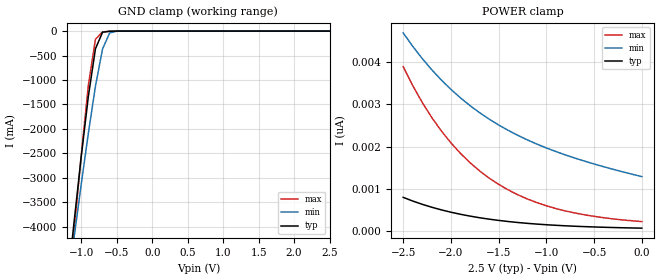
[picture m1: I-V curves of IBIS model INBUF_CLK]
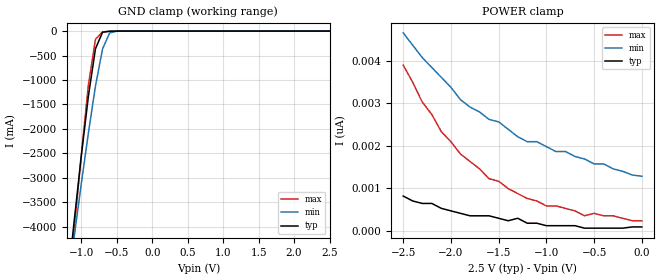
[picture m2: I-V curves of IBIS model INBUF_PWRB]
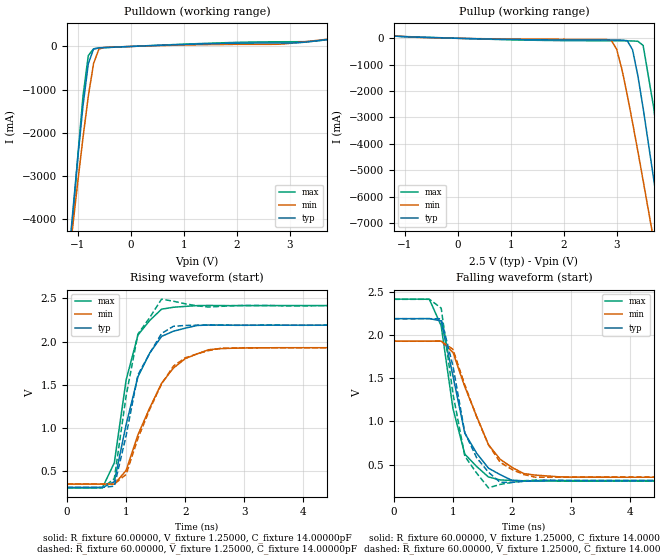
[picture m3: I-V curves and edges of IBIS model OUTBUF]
| IBIS file cspt857_mlf_2p5.ibs created by s2ibis2 version 1.2
| North Carolina State University Electronics Research Laboratory  1995
[IBIS ver]   2.1
[File name]   cspt857c_mlf_2p5.ibs
[File Rev]   1.0
[Date]   Friday, May 09, 2003
[Source]   IDT
[Notes]   1. Temp typ=25C, min=0C, max=100C
   2. IDT's 2.0v C11.5 process
   3. Ramp rate based on 50 ohm load
READ THESE TERMS AND CONDITIONS CAREFULLY BEFORE USING THIS IBIS MODEL.  BY
USING THIS IBIS MODEL, YOU ARE ACCEPTING AND AGREEING TO THESE TERMS AND
CONDITIONS OF USE.
Integrated Device Technology, Inc. ("IDT") hereby grants the user of this
IBIS model ("User") a non-exclusive, nontransferable license to use this
IBIS model under the following terms: The User is granted this license only
to use the IBIS model for demonstration purposes only and is not granted
rights to sell, copy (except as needed to run the IBIS model), rent, lease
or sub-license (except for demonstration) the IBIS model in whole or in
part, or in modified form to anyone. The User may modify the IBIS model to
suit its specific applications, but  rights to derivative works and such
modifications shall belong to IDT.
THIS IBIS MODEL IS PROVIDED ON AN AS IS" BASIS AND IDT  MAKES ABSOLUTELY NO
WARRANTY WITH RESPECT TO THE INFORMATION CONTAINED HEREIN.  IDT DISCLAIMS
AND USER WAIVES ALL WARRANTIES, EXPRESS AND IMPLIED, INCLUDING WARRANTIES OF
MERCHANTABILITY AND FITNESS FOR A PARTICULAR PURPOSE.  THE ENTIRE RISK AS TO
QUALITY AND PERFORMANCE IS WITH THE USER  ACCORDINGLY, IN NO EVENT SHALL IDT
BE LIABLE FOR ANY DIRECT OR INDIRECT DAMAGES, WHETHER IN CONTRACT OR TORT,
INCLUDING ANY LOST PROFITS OR OTHER INCIDENTAL, CONSEQUENTIAL, EXEMPLARY, OR
PUNITIVE DAMAGES ARISING OUT OF THE USE OR APPLICATION OF THE  IBIS MODEL,
WHETHER OR NOT IDT HAD NOTICE OF SUCH DAMAGES.
IDT reserves the right to make changes without notice to any product herein
to improve
reliability, function, or design. IDT does not convey any license under
patent rights or any other intellectual property rights, including those of
third parties. IDT is not obligated
to provide maintenance or support for the licensed IBIS model.
This model is for the 2.5V Phase Locked Loop Differential 1:10 SDRAM Clock
Driver
[Copyright]
Copyright 2002, Integrated Device Technology, Inc. All rights reserved.
|   Component CPST857C
[Component]   CPST857C
[Manufacturer]   Integrated Device Technology Inc.
[Package]
| variable   typ   min   max
R_pkg   86.00000m   61.00000m   0.11300
L_pkg   2.10000nH   1.50000nH   2.70000nH
C_pkg   0.20000pF   0.16000pF   0.24000pF
[Pin]  signal_name   model_name   R_pin   L_pin   C_pin
1   GND   GND
2   _Y2_   OUTBUF
3   Y2   OUTBUF
4   VDDQ   POWER
5   CLK   INBUF_CLK
6   _CLK_   INBUF_CLK
7   VDDQ   POWER
8   AVDD   POWER
9   AGND   GND
10   GND   GND
11   _Y3_   OUTBUF
12   Y3   OUTBUF
13   VDDQ   POWER
14   Y4   OUTBUF
15   _Y4_   OUTBUF
16   _Y9_   OUTBUF
17   Y9   OUTBUF
18   VDDQ   POWER
19   Y8   OUTBUF
20   _Y8_   OUTBUF
21   FBOUT   OUTBUF
22   _FBOUT_   OUTBUF
23   VDDQ   POWER
24   VDDQ   POWER
25   _FBIN_   INBUF_FBIN
26   FBIN   INBUF_FBIN
27   _PWRDWN_   INBUF_PWRB
28   VDDQ   POWER
29   Y7   OUTBUF
30   _Y7_   OUTBUF
31   _Y6_   OUTBUF
32   Y6   OUTBUF
33   VDDQ   POWER
34   Y5   OUTBUF
35   _Y5_   OUTBUF
36   _Y0_   OUTBUF
37   Y0   OUTBUF
38   VDDQ   POWER
39   Y1   OUTBUF
40   _Y1_   OUTBUF
| in   in   dummy_model
[Diff Pin]  inv_pin  vdiff   tdelay_typ  tdelay_min  tdelay_max
5   6   1.00000V  NA  |CLK<P:N> Clock Input  Pair
26   25   1.00000V  NA  |FBIN<P:N> FBIN Input  Pair
3   2   0.000V   NA  |Y2<P:N> Ouput  Pair
12   11   0.000V   NA  |Y3<P:N> Ouput  Pair
14   15   0.000V   NA  |Y4<P:N> Ouput  Pair
17   16   0.000V   NA  |Y9<P:N> Ouput  Pair
19   20   0.000V   NA  |Y8<P:N> Ouput  Pair
21   22   0.000V   NA  |FBOUT<P:N> Ouput  Pair
29   30   0.000V   NA  |Y7<P:N> Ouput  Pair
32   31   0.000V   NA  |Y6<P:N> Ouput  Pair
34   35   0.000V   NA  |Y5<P:N> Ouput  Pair
37   36   0.000V   NA  |Y0<P:N> Ouput  Pair
39   40   0.000V   NA  |Y1<P:N> Ouput  Pair
| Models and submodels in the file (4): INBUF_CLK (Input), INBUF_PWRB (Input), INBUF_FBIN (Input), OUTBUF (Output)
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|   Model INBUF_CLK
[Model]   INBUF_CLK
Model_type   Input
Polarity   Non-Inverting
Vinl =  0.80000V
Vinh =  2.00000V
C_comp   3.50000pF   3.50000pF   3.50000pF
[Temperature Range]   25.00000   100.00000   0.000
[Voltage Range]   2.50000V   2.30000V   2.70000V
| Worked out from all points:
|   GND clamp passes 1 mA (typ) near -0.52 V on its own axis
[GND_clamp]
| voltage   I(typ)   I(min)   I(max)
-2.5V     -23.89A    -20.36A    -27.98A
-1.2V     -5.248A    -5.316A    -5.713A
-1.1V     -3.884A    -4.209A    -4.089A
-1V       -2.564A    -3.127A    -2.526A
-900mV    -1.335A    -2.086A    -1.108A
-800mV    -361.3mA   -1.127A    -168.2mA
-700mV    -23.9mA    -365.3mA   -14.69mA
-600mV    -2.784mA   -39.09mA   -5.291mA
-500mV    -459.2uA   -2.159mA   -1.358mA
2.5V      71.27pA    1.402nA    195.1pA
[POWER_clamp]
| voltage   I(typ)   I(min)   I(max)
-2.5V     798.8pA    4.684nA    3.887nA
-2.4V     712pA      4.366nA    3.439nA
-2.3V     634.4pA    4.076nA    3.039nA
-2.2V     565pA      3.811nA    2.683nA
-2V       448.2pA    3.35nA     2.086nA
-1.8V     356pA      2.967nA    1.618nA
-1.7V     317.8pA    2.8nA      1.425nA
-1.5V     254.3pA    2.509nA    1.106nA
-1.2V     185.1pA    2.157nA    761.7pA
-900mV    138.7pA    1.881nA    534.7pA
-500mV    99.57pA    1.587nA    349.9pA
0V        71.27pA    1.288nA    226.3pA
|   Model INBUF_PWRB
[Model]   INBUF_PWRB
Model_type   Input
Polarity   Non-Inverting
Vinl =  0.80000V
Vinh =  2.00000V
C_comp   3.50000pF   3.50000pF   3.50000pF
[Temperature Range]   25.00000   100.00000   0.000
[Voltage Range]   2.50000V   2.30000V   2.70000V
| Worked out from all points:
|   GND clamp passes 1 mA (typ) near -0.52 V on its own axis
[GND_clamp]
| voltage   I(typ)   I(min)   I(max)
-2.5V     -23.88A    -20.35A    -27.98A
-1.2V     -5.247A    -5.316A    -5.712A
-1.1V     -3.884A    -4.209A    -4.088A
-1V       -2.564A    -3.127A    -2.526A
-900mV    -1.335A    -2.086A    -1.108A
-800mV    -361.3mA   -1.126A    -168.2mA
-700mV    -23.9mA    -365.3mA   -14.69mA
-600mV    -2.784mA   -39.09mA   -5.291mA
-500mV    -459.2uA   -2.159mA   -1.358mA
2.5V      87.31pA    1.397nA    232.8pA
[POWER_clamp]
| voltage   I(typ)   I(min)   I(max)
-2.5V     814.9pA    4.657nA    3.9nA
-2.3V     640.3pA    4.075nA    3.027nA
-2.1V     523.9pA    3.609nA    2.328nA
-1.9V     407.5pA    3.085nA    1.804nA
-1.6V     349.2pA    2.619nA    1.222nA
-1.5V     291pA      2.561nA    1.164nA
-1.3V     291pA      2.212nA    873.1pA
-1.2V     174.6pA    2.095nA    756.7pA
-1V       116.4pA    1.979nA    582.1pA
-600mV    58.21pA    1.688nA    349.2pA
-500mV    58.21pA    1.572nA    407.5pA
0V        87.31pA    1.281nA    232.8pA
|   Model OUTBUF
[Model]   OUTBUF
Model_type   Output
Polarity   Non-Inverting
Vmeas =  1.25000V
C_comp   3.50000pF   3.50000pF   3.50000pF
[Temperature Range]   25.00000   100.00000   0.000
[Voltage Range]   2.50000V   2.30000V   2.70000V
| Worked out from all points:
|   slope of the pulldown table from 0 to 0.375 V, typ, clamps not added: 20.3 ohm
|   slope of the pullup table from 0 to 0.375 V, typ, clamps not added: 20 ohm
|   rising waveform, R_fixture 60.00000, V_fixture 1.25000, C_fixture 14.00000pF: 20-80 % time 468ps typ, 633ps min, 341ps max; typ from 0.315 V to 2.19 V
|   rising waveform, R_fixture 60.00000, V_fixture 1.25000, C_fixture 14.00000pF: 20-80 % time 436ps typ, 602ps min, 308ps max; typ from 0.316 V to 2.19 V
|   falling waveform, R_fixture 60.00000, V_fixture 1.25000, C_fixture 14.00000pF: 20-80 % time 441ps typ, 581ps min, 335ps max; typ from 2.19 V to 0.315 V
|   falling waveform, R_fixture 60.00000, V_fixture 1.25000, C_fixture 14.00000pF: 20-80 % time 388ps typ, 552ps min, 299ps max; typ from 2.19 V to 0.316 V
[Pulldown]
| voltage   I(typ)   I(min)   I(max)
-2.5V     -24.02A    -20.48A    -28.11A
-1.3V     -6.698A    -6.489A    -7.44A
-1.1V     -3.936A    -4.25A     -4.147A
-1V       -2.612A    -3.164A    -2.58A
-900mV    -1.378A    -2.12A     -1.157A
-800mV    -400.3mA   -1.157A    -211.8mA
-700mV    -58.29mA   -391.9mA   -53.12mA
-600mV    -32.51mA   -62.11mA   -38.49mA
-500mV    -25.4mA    -21.54mA   -29.24mA
2.8V      81.34mA    52.63mA    108.7mA
3.2V      89.68mA    97.53mA    110.8mA
5V        376.9mA    361.1mA    377.2mA
[Pullup]
| voltage   I(typ)   I(min)   I(max)
-2.5V     286.8mA    273.7mA    294mA
-900mV    50.69mA    50.88mA    59.76mA
2.9V      -64.27mA   -81.77mA   -93.6mA
3V        -64.95mA   -412.9mA   -93.85mA
3.2V      -91.83mA   -2.145A    -95.98mA
3.3V      -434.2mA   -3.192A    -101.2mA
3.4V      -1.414A    -4.28A     -112.7mA
3.5V      -2.65A     -5.394A    -270mA
3.7V      -5.347A    -7.664A    -2.64A
3.9V      -8.156A    -9.969A    -5.841A
4.1V      -11.01A    -12.29A    -9.193A
5V        -24.08A    -22.88A    -24.72A
[Ramp]
| variable   typ   min   max
dV/dt_r   1.04760/0.15068n   0.82920/0.17415n   1.21080/0.13672n
dV/dt_f   1.05510/0.13771n   0.87414/0.16331n   1.18398/0.13634n
R_load = 50.00000
[Rising Waveform]
R_fixture = 60.00000
V_fixture = 1.25000
V_fixture_min = 1.15000
V_fixture_max = 1.35000
C_fixture = 14.00000pF
| time   V(typ)   V(min)   V(max)
0s        315.1mV    354mV      310.2mV
600ps     314.6mV    354mV      313.6mV
800ps     380.5mV    352.7mV    599.6mV
1ns       1.042V     511.7mV    1.557V
1.2ns     1.595V     922.9mV    2.076V
1.4ns     1.869V     1.235V     2.245V
1.6ns     2.061V     1.518V     2.376V
2ns       2.155V     1.803V     2.408V
2.6ns     2.192V     1.919V     2.417V
10ns      2.191V     1.93V      2.417V
[Rising Waveform]
R_fixture = 60.00000
V_fixture = 1.25000
V_fixture_min = 1.15000
V_fixture_max = 1.35000
C_fixture = 14.00000pF
R_dut = 86.00000m
L_dut = 2.10000nH
C_dut = 0.20000pF
| time   V(typ)   V(min)   V(max)
0s        316.1mV    354.8mV    311.4mV
600ps     316mV      354.8mV    311.4mV
800ps     329.3mV    354.3mV    416.1mV
1ns       913.4mV    465.2mV    1.374V
1.2ns     1.617V     881.1mV    2.088V
1.6ns     2.095V     1.51V      2.491V
1.8ns     2.178V     1.718V     2.467V
2ns       2.187V     1.812V     2.438V
2.6ns     2.192V     1.923V     2.408V
10ns      2.19V      1.929V     2.415V
[Falling Waveform]
R_fixture = 60.00000
V_fixture = 1.25000
V_fixture_min = 1.15000
V_fixture_max = 1.35000
C_fixture = 14.00000pF
| time   V(typ)   V(min)   V(max)
0s        2.191V     1.93V      2.417V
600ps     2.192V     1.93V      2.415V
800ps     2.164V     1.931V     2.108V
1ns       1.526V     1.799V     1.147V
1.2ns     864.3mV    1.401V     621.2mV
1.6ns     459.2mV    731.7mV    356.9mV
1.8ns     383.4mV    560.5mV    322.2mV
2.2ns     311.3mV    396mV      312.7mV
2.8ns     315.2mV    358.3mV    310.2mV
10ns      315.1mV    354mV      310.2mV
[Falling Waveform]
R_fixture = 60.00000
V_fixture = 1.25000
V_fixture_min = 1.15000
V_fixture_max = 1.35000
C_fixture = 14.00000pF
R_dut = 86.00000m
L_dut = 2.10000nH
C_dut = 0.20000pF
| time   V(typ)   V(min)   V(max)
0s        2.19V      1.929V     2.415V
600ps     2.19V      1.929V     2.415V
800ps     2.189V     1.93V      2.313V
1ns       1.639V     1.835V     1.319V
1.2ns     870.2mV    1.424V     597.9mV
1.4ns     580.4mV    1.054V     402.2mV
1.6ns     412mV      730.6mV    230.6mV
1.8ns     293.9mV    526.2mV    270.9mV
2.4ns     313.9mV    353.2mV    320.4mV
10ns      316.1mV    354.8mV    311.4mV
